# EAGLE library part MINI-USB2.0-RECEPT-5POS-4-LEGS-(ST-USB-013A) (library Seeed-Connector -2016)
320010014
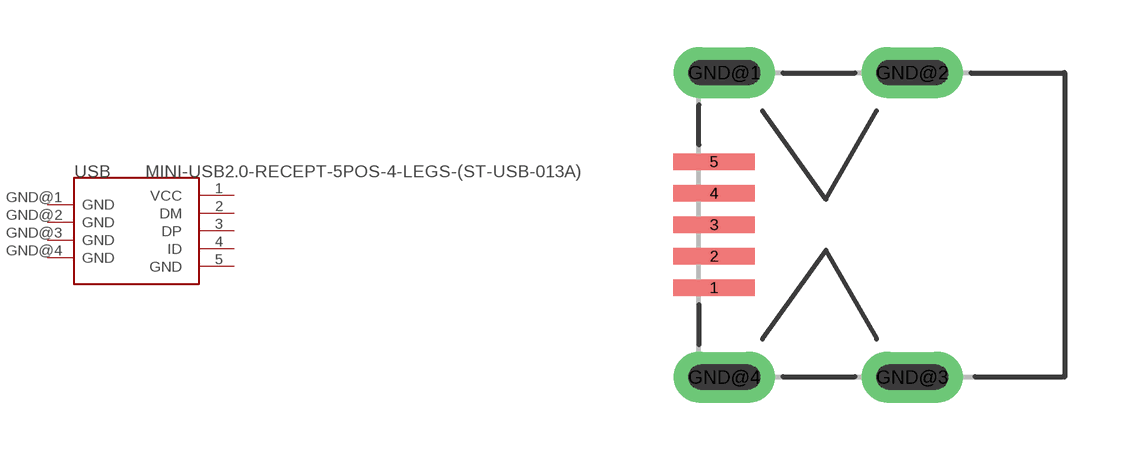
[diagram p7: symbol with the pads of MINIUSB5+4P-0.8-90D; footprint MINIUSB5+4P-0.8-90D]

Designator prefix USB

## MINI-USB2.0-RECEPT-5POS-4-LEGS-(ST-USB-013A) (MPN: ST-USB-013A; VALUE: ST-USB-013A)  [MINIUSB5+4P-0.8-90D]
1  VCC
2  DM
3  DP
4  ID
5  GND
GND@1  GND
GND@2  GND
GND@3  GND
GND@4  GND

## Footprint MINIUSB5+4P-0.8-90D (pad centres in mm)
smd 2.032 x 0.406: 1 0.381,-1.575; 2 0.381,-0.787; 3 0.381,0; 4 0.381,0.787; 5 0.381,1.575
drill 0.635 pad 1.27 long: GND@1 0.635,3.81; GND@2 5.334,3.81; GND@3 5.334,-3.81; GND@4 0.635,-3.81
